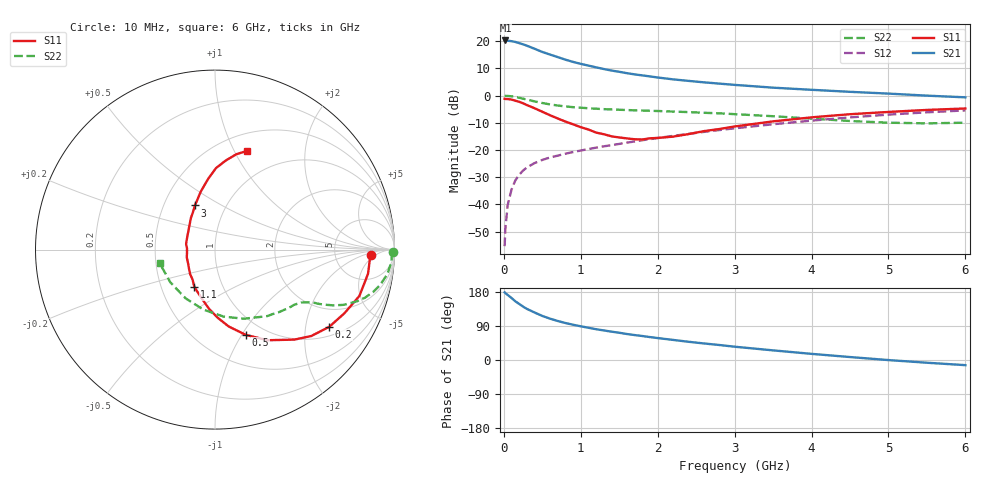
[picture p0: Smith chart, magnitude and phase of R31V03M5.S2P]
! SIEMENS Small Signal Semiconductors
! BFR181
! Si NPN RF Bipolar Junction Transistor in SOT23
! VCE = 1 V  IC = 3.5 mA
! Common Emitter S-Parameters:  May  1996
# GHz  S  MA  R  50
!  f  S11  S21  S12  S22
! GHz  MAG  ANG  MAG  ANG  MAG  ANG  MAG  ANG
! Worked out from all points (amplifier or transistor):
!   36 points, 10 MHz to 6 GHz, reference 50 ohm
!   highest |S21| = 20.3 dB at 20 MHz (marker M1)
!   |S21| within 3 dB of that: start of sweep to 394.4 MHz
!   unconditionally stable (mu >= 1): 1.172 GHz to 3.287 GHz
!   at 250 MHz: K = 0.35, MSG = 23.2 dB, |S12| = -27.6 dB
!   at 1.4 GHz: K = 1.06, MAG = 12.2 dB, |S12| = -18.2 dB
!   at 6 GHz: K = 0.89, MSG = 2.4 dB, |S12| = -5.5 dB
!   S11 on the Smith chart (normalised r, x): 10 MHz: 14, -3; 200 MHz: 1.29, -2.71; 500 MHz: 0.82, -1.04; 1.1 GHz: 0.73, -0.32; 3 GHz: 0.71, +0.38; 6 GHz: 0.68, +1.13
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0.01  0.8707 -1.8  10.23 178.5  0.0017 86.7  0.9911 -0.8
0.02  0.8645 -3.5  10.32 176.5  0.0036 90.0  0.9859 -1.7
0.05  0.8632 -9.0  10.22 171.6  0.0097 85.4  0.9849 -4.2
0.1  0.8449 -17.8  9.999 163.7  0.0187 79.5  0.9693 -8.2
0.15  0.8035 -26.2  9.685 154.8  0.0277 75.1  0.9408 -12.1
0.2  0.7681 -34.1  9.215 148.0  0.035 72.0  0.9112 -15.1
0.25  0.7208 -41.9  8.76 140.9  0.0418 68.3  0.8772 -17.8
0.3  0.6685 -48.6  8.264 134.8  0.0477 66.3  0.8423 -20.0
0.4  0.5837 -59.9  7.252 125.3  0.0574 61.8  0.7811 -23.2
0.5  0.5046 -70.2  6.338 116.3  0.0656 59.8  0.73 -25.2
0.6  0.4351 -79.9  5.679 109.1  0.0727 58.2  0.6886 -26.5
0.7  0.3789 -87.9  5.1 103.0  0.0786 57.8  0.6559 -27.5
0.8  0.3331 -95.5  4.579 97.6  0.0852 57.3  0.631 -28.1
1.1  0.2374 -119.0  3.557 85.1  0.1039 57.7  0.5846 -30.2
1.3  0.1947 -135.4  3.077 78.0  0.1166 58.3  0.5632 -31.6
1.6  0.1631 -164.4  2.58 68.6  0.1364 58.9  0.5424 -34.3
2.2  0.1757 149.1  1.987 53.0  0.1815 58.4  0.508 -41.8
3  0.2701 114.5  1.573 35.1  0.2499 54.6  0.4553 -55.3
3.5  0.3354 103.4  1.398 25.4  0.297 50.7  0.4172 -67.4
4.5  0.4541 89.3  1.172 7.8  0.3967 40.4  0.3407 -100.9
5.5  0.5444 77.4  0.997 -7.2  0.4922 27.6  0.3084 -143.9
6  0.5787 72.0  0.928 -13.6  0.5339 20.4  0.3172 -166.0
